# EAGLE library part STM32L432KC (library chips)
Simple STM32 Cortex M4. Features include a fast 32bit timer, 2 spi, 2 i2c, 2usart, hardware aes and more.
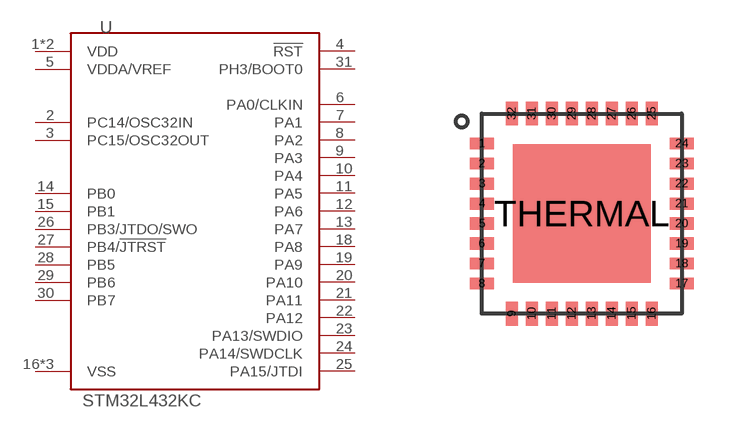
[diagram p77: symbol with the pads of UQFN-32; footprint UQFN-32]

Designator prefix U

## STM32L432KC (DIGIKEY: 497-16578-ND; MANUFACTURER: STMicroelectronics; MPN: STM32L432KCU6)  [UQFN-32]
1  VDD
2  PC14/OSC32IN
3  PC15/OSC32OUT
4  !RST
5  VDDA/VREF
6  PA0/CLKIN
7  PA1
8  PA2
9  PA3
10  PA4
11  PA5
12  PA6
13  PA7
14  PB0
15  PB1
16  VSS
17  VDD
18  PA8
19  PA9
20  PA10
21  PA11
22  PA12
23  PA13/SWDIO
24  PA14/SWDCLK
25  PA15/JTDI
26  PB3/JTDO/SWO
27  PB4/!JTRST
28  PB5
29  PB6
30  PB7
31  PH3/BOOT0
32  VSS
THERMAL  VSS

## Footprint UQFN-32 (pad centres in mm)
smd 0.6 x 0.3: 1 -2.5,1.75; 2 -2.5,1.25; 3 -2.5,0.75; 4 -2.5,0.25; 5 -2.5,-0.25; 6 -2.5,-0.75; 7 -2.5,-1.25; 8 -2.5,-1.75; 17 2.5,-1.75; 18 2.5,-1.25; 19 2.5,-0.75; 20 2.5,-0.25; 21 2.5,0.25; 22 2.5,0.75; 23 2.5,1.25; 24 2.5,1.75
smd 0.3 x 0.6: 9 -1.75,-2.5; 10 -1.25,-2.5; 11 -0.75,-2.5; 12 -0.25,-2.5; 13 0.25,-2.5; 14 0.75,-2.5; 15 1.25,-2.5; 16 1.75,-2.5; 25 1.75,2.5; 26 1.25,2.5; 27 0.75,2.5; 28 0.25,2.5; 29 -0.25,2.5; 30 -0.75,2.5; 31 -1.25,2.5; 32 -1.75,2.5
smd 3.45 x 3.45: THERMAL 0,0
